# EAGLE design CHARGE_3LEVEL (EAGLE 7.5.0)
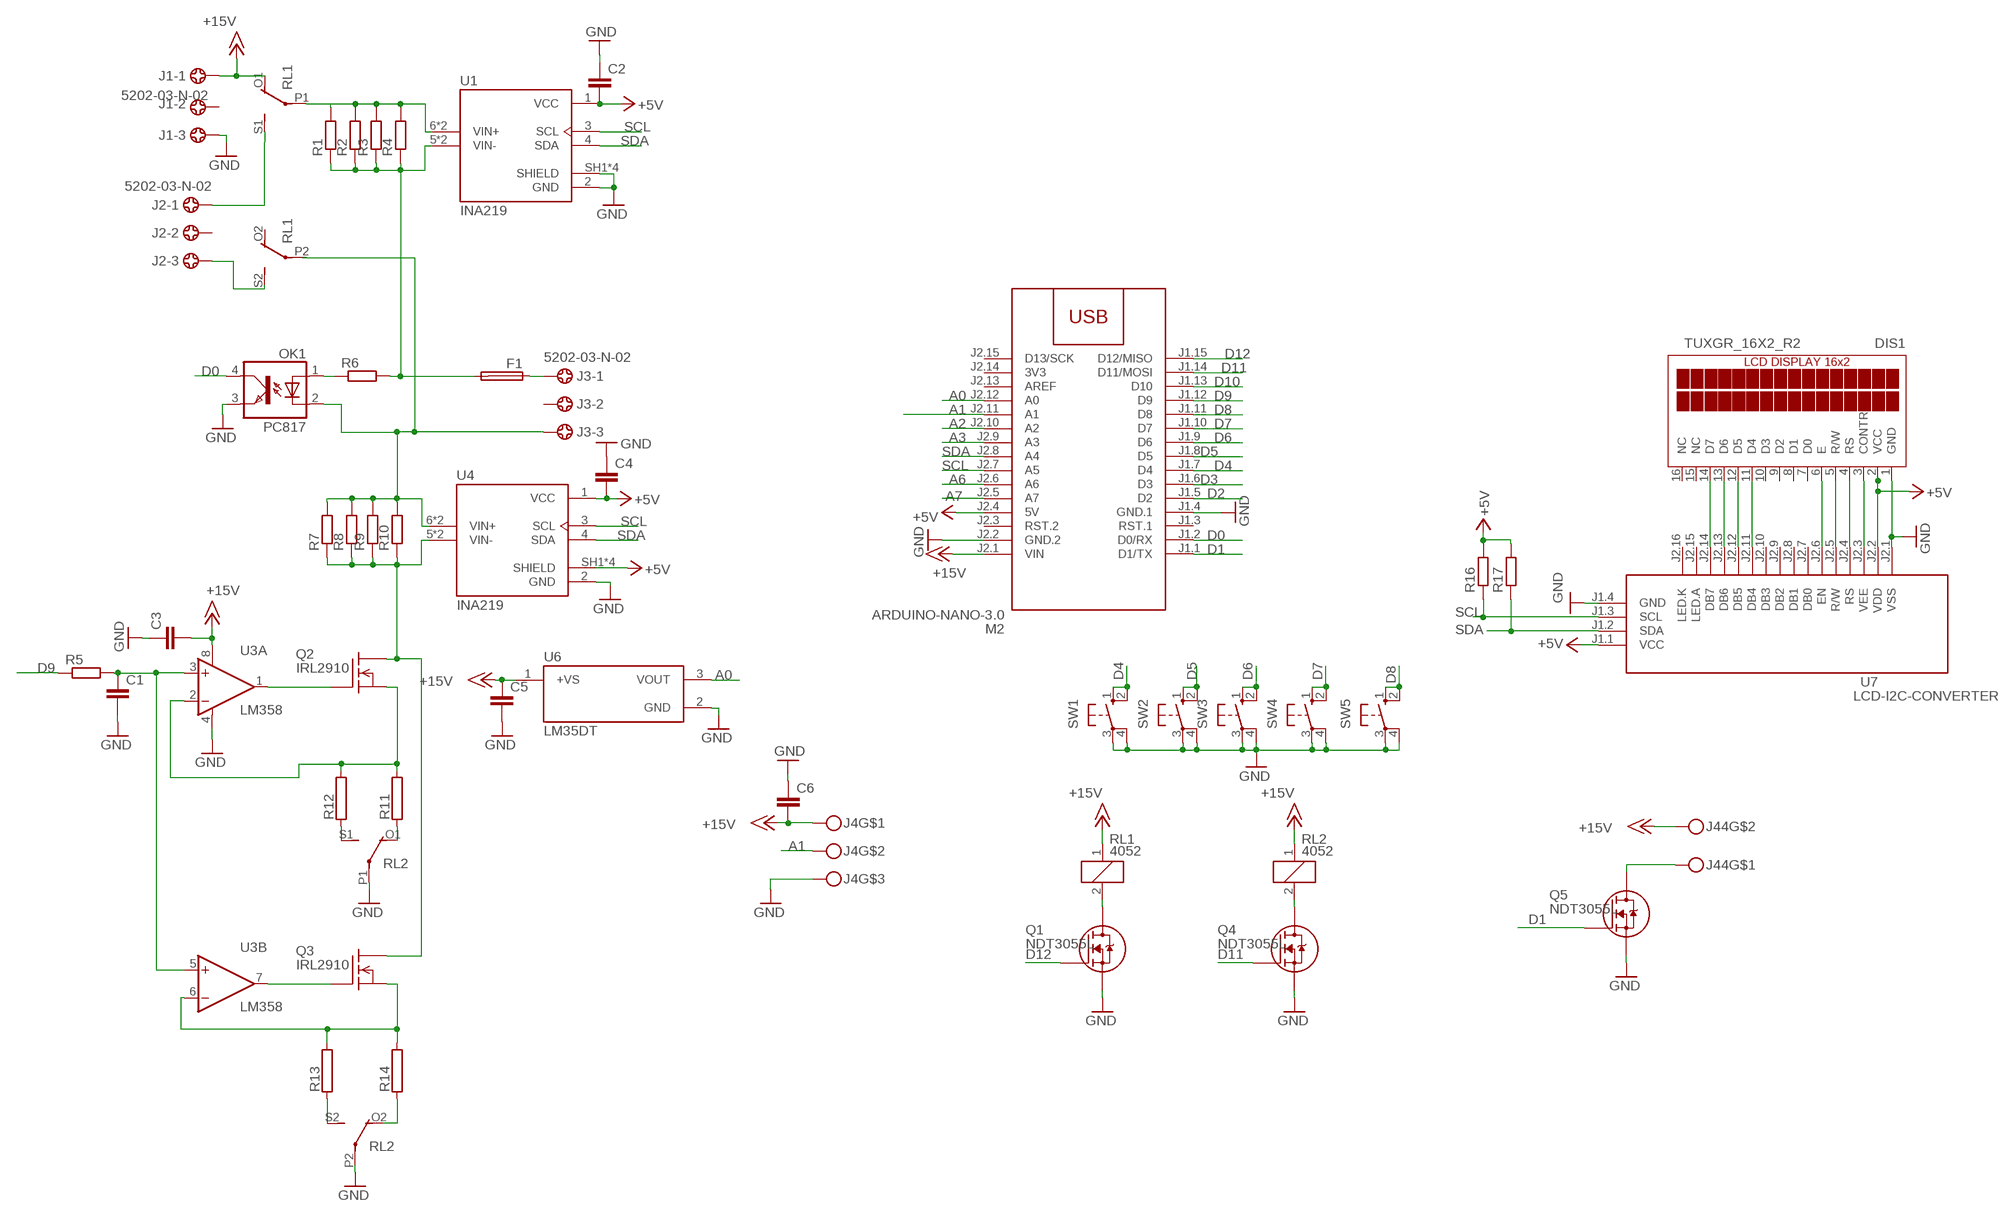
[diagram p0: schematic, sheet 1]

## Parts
C1  C-EUC1206  [C1206]
C2  C-EUC1206  [C1206]
C3  C-EUC1206  [C1206]
C4  C-EUC1206  [C1206]
C5  C-EUC1206  [C1206]
C6  C-EUC1206  [C1206]
DIS1  TUXGR_16X2_R2  [TUXGR_16X2_R2]
F1  FUSEBLANK_5X20MM  [FUSE_HOLDER_5X20MM]
J1  5202-03-N-02  [5202-03-N-02]
J2  5202-03-N-02  [5202-03-N-02]
J3  5202-03-N-02  [5202-03-N-02]
J4  MKDSN3  [MKDSN3]
J44  MKDSN1,5-2-5,08  [MKDSN1,5-2-5,08]
M2  ARDUINO-NANO-3.0  [ARDUINO-NANO-3.0]
OK1  PC817  [DIL04]
Q1  NDT3055L  [SOT223-4]
Q2  IRL2910  IRF540  [TO220]
Q3  IRL2910  IRF540  [TO220]
Q4  NDT3055L  [SOT223-4]
Q5  NDT3055L  [SOT223-4]
R1  R-EU_R2512  [R2512]
R2  R-EU_R2512  [R2512]
R3  R-EU_R2512  [R2512]
R4  R-EU_R2512  [R2512]
R5  R-EU_R1206  [R1206]
R6  R-EU_R1206  [R1206]
R7  R-EU_R2512  [R2512]
R8  R-EU_R2512  [R2512]
R9  R-EU_R2512  [R2512]
R10  R-EU_R2512  [R2512]
R11  RCA4200  [CA4200]
R12  RAC07  [AC07]
R13  RAC07  [AC07]
R14  RCA4200  [CA4200]
R16  R-EU_R1206  [R1206]
R17  R-EU_R1206  [R1206]
RL1  4052  [F4052]
RL2  4052  [F4052]
SW1  40-XX  [B3F-40XX]
SW2  40-XX  [B3F-40XX]
SW3  40-XX  [B3F-40XX]
SW4  40-XX  [B3F-40XX]
SW5  40-XX  [B3F-40XX]
U1  INA219  [MODULE_INA219]
U3  LM358  OPA2234U  [SO08]
U4  INA219  [MODULE_INA219]
U6  LM35DT  [TO254P1016X457X1955-3]
U7  LCD-I2C-CONVERTER  [LCD-I2C-CONVERTER]

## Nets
+5V: C2.2 C4.2 DIS1.2(VCC) M2.J2.4(5V) R16.2 R17.2 U1.1(VCC) U4.1(VCC) U4.SH1(SHIELD) U4.SH2(SHIELD) U4.SH3(SHIELD) U4.SH4(SHIELD) U7.J1.1(VCC) U7.J2.2(VDD)
+15V: C3.2 C5.1 C6.2 J1.1 J4.1 J44.2 M2.J2.1(VIN) RL1.1 RL1.O1(2:O) RL2.1 U3.8(A:V+) U6.1(+VS)
A0: M2.J2.12(A0) U6.3(VOUT)
A1: J4.2 M2.J2.11(A1)
A2: M2.J2.10(A2)
A3: M2.J2.9(A3)
A6: M2.J2.6(A6)
A7: M2.J2.5(A7)
D0: M2.J1.2(D0/RX) OK1.4(COL)
D1: M2.J1.1(D1/TX) Q5.1(G)
D2: M2.J1.5(D2)
D3: M2.J1.6(D3)
D4: M2.J1.7(D4) SW1.1(S) SW1.2(S1)
D5: M2.J1.8(D5) SW2.1(S) SW2.2(S1)
D6: M2.J1.9(D6) SW3.1(S) SW3.2(S1)
D7: M2.J1.10(D7) SW4.1(S) SW4.2(S1)
D8: M2.J1.11(D8) SW5.1(S) SW5.2(S1)
D9: M2.J1.12(D9) R5.1
D10: M2.J1.13(D10)
D11: M2.J1.14(D11/MOSI) Q4.1(G)
D12: M2.J1.15(D12/MISO) Q1.1(G)
GND: C1.2 C2.1 C3.1 C4.1 C5.2 C6.1 DIS1.1(GND) J1.3 J4.3 M2.J1.4(GND.1) M2.J2.2(GND.2) OK1.3(EMIT) Q1.3(S) Q4.3(S) Q5.3(S) RL2.P1(2:P) RL2.P2(3:P) SW1.3(P) SW1.4(P1) SW2.3(P) SW2.4(P1) SW3.3(P) SW3.4(P1) SW4.3(P) SW4.4(P1) SW5.3(P) SW5.4(P1) U1.2(GND) U1.SH1(SHIELD) U1.SH2(SHIELD) U1.SH3(SHIELD) U1.SH4(SHIELD) U3.4(A:V-) U4.2(GND) U6.2(GND) U7.J1.4(GND) U7.J2.1(VSS)
N$1: DIS1.14(D7) U7.J2.14(DB7)
N$2: DIS1.13(D6) U7.J2.13(DB6)
N$3: DIS1.12(D5) U7.J2.12(DB5)
N$4: DIS1.11(D4) U7.J2.11(DB4)
N$5: DIS1.6(E) U7.J2.6(EN)
N$6: DIS1.5(R/W) U7.J2.5(R/W)
N$7: DIS1.4(RS) U7.J2.4(RS)
N$8: Q2.1(G) U3.1(A:OUT)
N$9: F1.2 R1.1 R2.1 R3.1 R4.1 R6.2 U1.5(VIN-) U1.VIN-
N$10: DIS1.3(CONTR) U7.J2.3(VEE)
N$11: F1.1 J3.1
N$12: J3.3 OK1.2(C) R7.2 R8.2 R9.2 R10.2 U4.6(VIN+) U4.VIN+
N$13: OK1.1(A) R6.1
N$14: Q2.3(S) R11.2 R12.2 U3.2(A:-IN)
N$15: R13.1 RL2.S2(3:S)
N$16: Q2.2(D) Q3.2(D) R7.1 R8.1 R9.1 R10.1 U4.5(VIN-) U4.VIN-
N$17: Q3.1(G) U3.7(B:OUT)
N$18: J44.1 Q5.2(D) Q5.4(D)
N$19: C1.1 R5.2 U3.3(A:+IN) U3.5(B:+IN)
N$20: R1.2 R2.2 R3.2 R4.2 RL1.P1(2:P) U1.6(VIN+) U1.VIN+
N$21: R12.1 RL2.S1(2:S)
N$22: J2.1 RL1.S1(2:S)
N$23: J2.3 RL1.S2(3:S)
N$24: R11.1 RL2.O1(2:O)
N$25: Q3.3(S) R13.2 R14.2 U3.6(B:-IN)
N$26: R14.1 RL2.O2(3:O)
N$27: Q1.2(D) Q1.4(D) RL1.2
N$28: Q4.2(D) Q4.4(D) RL2.2
SCL: M2.J2.7(A5) R16.1 U1.3(SCL) U4.3(SCL) U7.J1.3(SCL)
SDA: M2.J2.8(A4) R17.1 U1.4(SDA) U4.4(SDA) U7.J1.2(SDA)
Unconnected: DIS1.7(D0) DIS1.8(D1) DIS1.9(D2) DIS1.10(D3) DIS1.15(NC) DIS1.16(NC) J1.2 J2.2 J3.2 M2.J1.3(RST.1) M2.J2.3(RST.2) M2.J2.13(AREF) M2.J2.15(D13/SCK) RL1.O2(3:O) RL1.P2(3:P) U7.J2.7(DB0) U7.J2.8(DB1) U7.J2.9(DB2) U7.J2.10(DB3) U7.J2.15(LED.A) U7.J2.16(LED.K)

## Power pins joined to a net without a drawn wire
3V3: M2.J2.14(3V3)

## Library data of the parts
C1-C6 = rcl:C-EU: CAPACITOR, European symbol
DIS1 = display-lcd:TUXGR_16X2_R2: Tuxgraphics LCD display 16x2 characters reflective, without background light Source: tuxgr_12x2_r2.pdf; OC_FARNELL: unknown; OC_NEWARK: unknown
F1 = fuse:FUSE: Fuse; OC_FARNELL: unknown; OC_NEWARK: unknown
J1-J3 = con-ebyelectro:5202-03-N-02: Barrier Blocks Sreies 5202 Source: http://www.ebyelectro.com/PDF/5202-XX-N-02.pdf; OC_FARNELL: unknown; OC_NEWARK: unknown
J4 = con-phoenix-508:MKDSN3
J44 = con-phoenix-508:MKDSN1,5-2-5,08
M2 = diy-modules:ARDUINO-NANO-3.0: Arduino Nano 3.0 and compatible devices More details available here: https://www.arduino.cc/en/Main/ArduinoBoardNano Click here to find device on ebay.com
OK1 = optocoupler:PC817: SHARP OPTO COUPLER; MPN: PC817X4J000F; OC_FARNELL: 9707727; OC_NEWARK: 97K7059
Q1 Q4 Q5 = NDT3055L:NDT3055L: Trans MOSFET N-CH 60V 4A 4-Pin(3+Tab) SOT-223 Trans MOSFET N-CH 60V 4A 4-Pin(3+Tab) SOT-223 Check availability; AVAILABILITY: In Stock; CHECK_PRICES: https://www.snapeda.com/parts/NDT3055L/Onsemi/view-part/?ref=eda; DESCRIPTION: Trans MOSFET N-CH 60V 4A 4-Pin(3+Tab) SOT-223 Trans MOSFET N-CH 60V 4A 4-Pin(3+Tab) SOT-223; MF: ON; MP: NDT3055L; PACKAGE: SOT-223-4 Fairchild Semiconductor; PRICE: None; SNAPEDA_LINK: https://www.snapeda.com/parts/NDT3055L/Onsemi/view-part/?ref=snap
Q2 Q3 = transistor-fet:IRF540: N-Channel Enhancement MOSFET (HEXFET); 100V; 28A; 0,077Ohm
R1-R10 R16 R17 = rcl:R-EU_: RESISTOR, European symbol
R11-R14 = resistor-power:R: Power Resitor; OC_FARNELL: unknown; OC_NEWARK: unknown
RL1 RL2 = relay:4052: RELAY 2 x switch, Finder; OC_FARNELL: unknown; OC_NEWARK: unknown
SW1-SW5 = switch-omron:40-XX: OMRON SWITCH; MF: OMRON COMPONENTS USA; MPN: B3F-4000; OC_FARNELL: 176434; OC_NEWARK: 36K3105
U1 U4 = INA219:INA219: Check availability; AVAILABILITY: Not in stock; CHECK_PRICES: https://www.snapeda.com/parts/INA219%20High%20Side%20DC%20Current%20Sensor%20Breakout%20-%2026V%20%C2%B13.2A%20Max%20-%20STEMMA%20QT/Adafruit+Industries/view-part/?ref=eda; DESCRIPTION: INA219 High Side DC Current Sensor Breakout - 26V ±3.2A Max | Adafruit Industries 904; MF: Adafruit Industries; MP: INA219 High Side DC Current Sensor Breakout - 26V ±3.2A Max - STEMMA QT; PACKAGE: NON-STANDARD-8 ADAFRUIT; PRICE: None; SNAPEDA_LINK: https://www.snapeda.com/parts/INA219%20High%20Side%20DC%20Current%20Sensor%20Breakout%20-%2026V%20%C2%B13.2A%20Max%20-%20STEMMA%20QT/Adafruit+Industries/view-part/?ref=snap
U3 = burr-brown:OPA2234: Operational Amplifier; MF: TEXAS INSTRUMENTS; MPN: OPA2234U; OC_FARNELL: 1212441; OC_NEWARK: 96K4523
U6 = LM35DT-H:LM35DT: Check availability; AVAILABILITY: In Stock; CHECK_PRICES: https://www.snapeda.com/parts/LM35DT/Texas+Instruments/view-part/?ref=eda; DESCRIPTION: ±0.5°C 4V-30V, Temperature sensor with analog output 3-TO-220 0 to 100; MF: Texas Instruments; MP: LM35DT; PACKAGE: TO-220-3 Texas Instruments; PRICE: None; SNAPEDA_LINK: https://www.snapeda.com/parts/LM35DT/Texas+Instruments/view-part/?ref=snap
U7 = diy-modules:LCD-I2C-CONVERTER: I2C Bus to 4-Bit Parallel LCD Interface with LED backlight driver

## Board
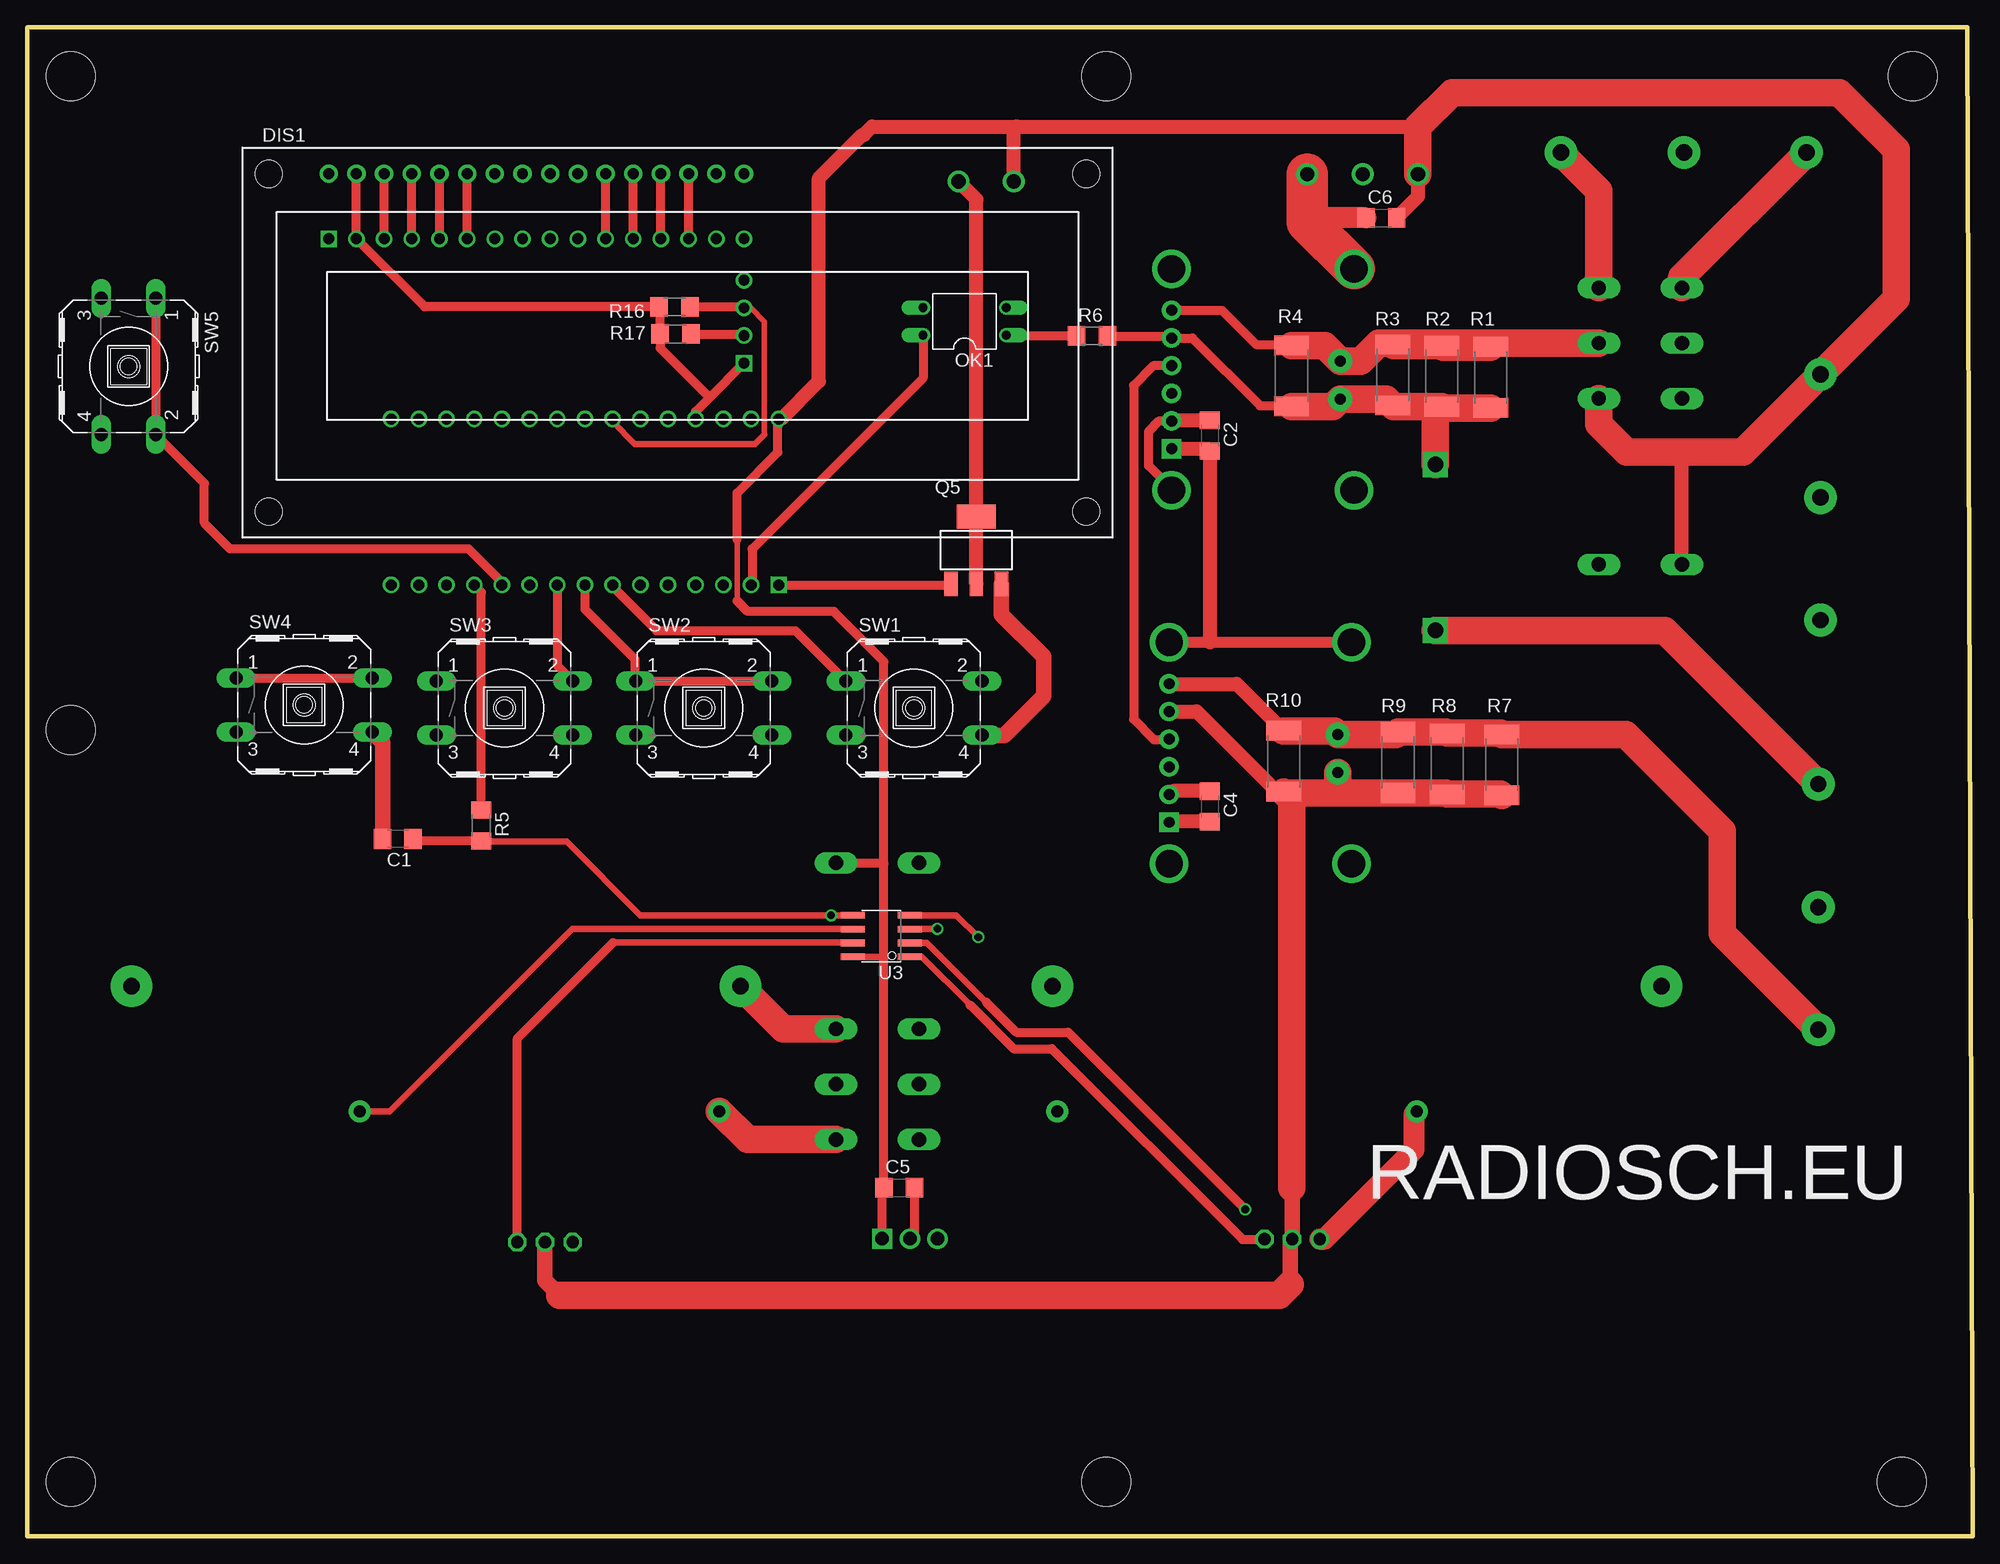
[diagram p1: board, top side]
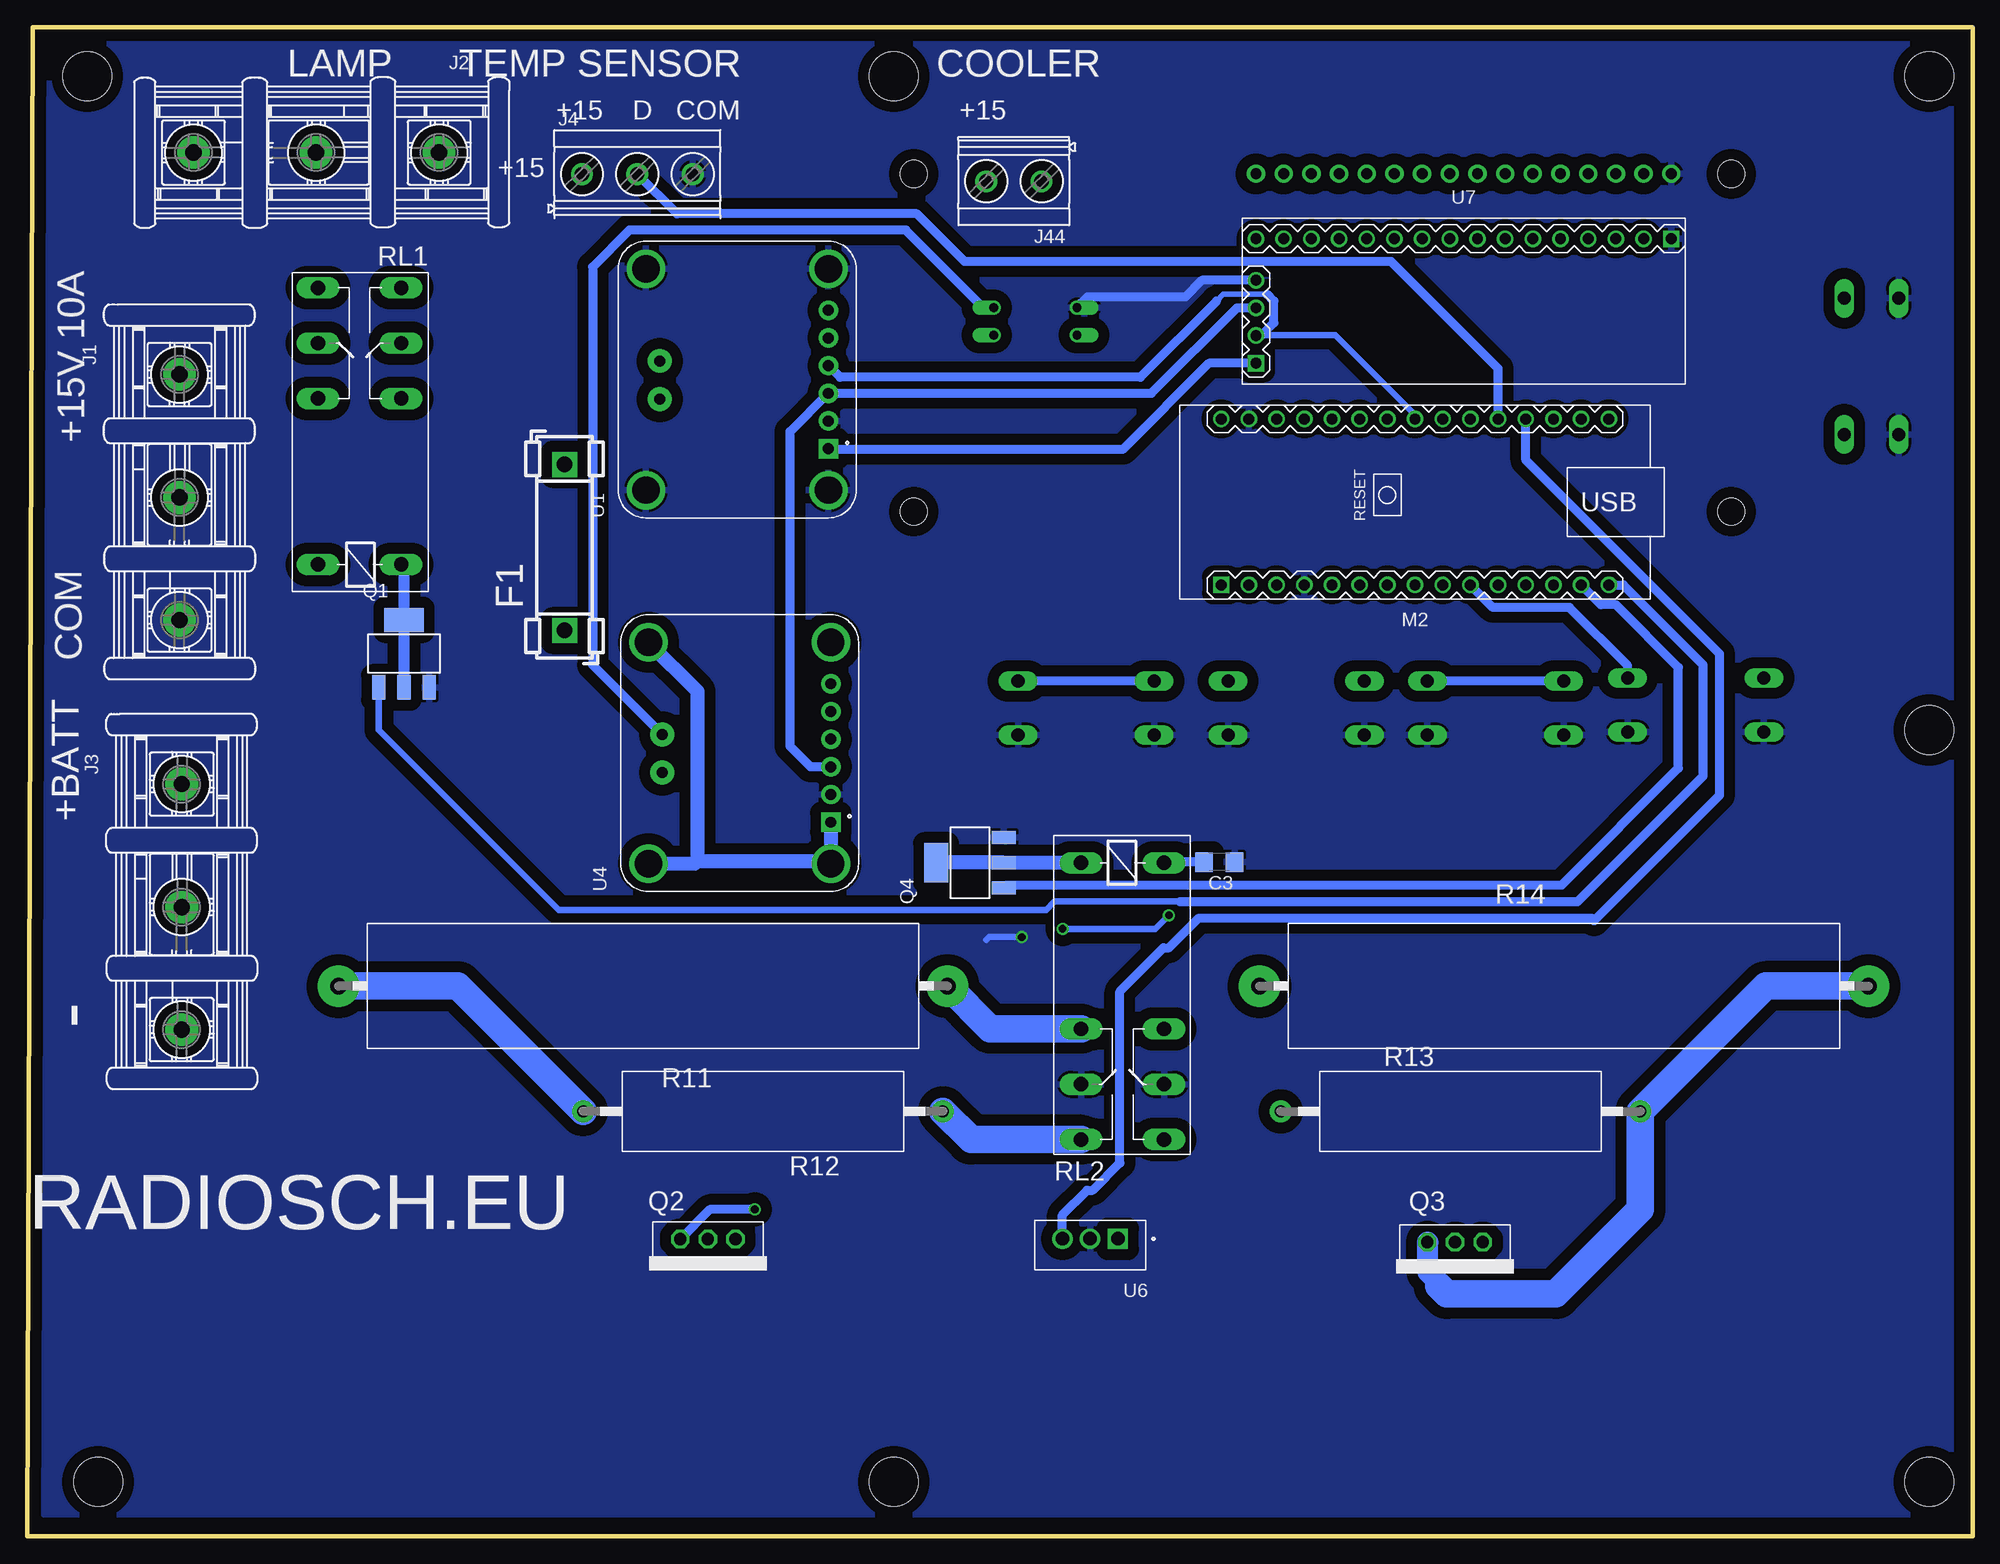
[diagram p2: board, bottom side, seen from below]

Size 178.5 x 138.5 mm. Coordinates in mm from the lower left corner, seen from the top.
Outline: 0,0 178.5,0 178,138.5 0,138.5 0,0
Copper layers (1*16): Top 0.035mm / dielectric 1.5mm / Bottom 0.035mm
Design rules "default": minimum track width 10mil, minimum drill 24mil, track to track 8mil, track to pad 8mil, pad to pad 8mil, via to via 8mil, smd to smd 8mil, copper to edge 40mil, drill to drill 8mil, minimum pad ring 10mil, minimum via ring 8mil, stop-mask expansion 4mil, vias tented up to drill 0mil, thermal gap 10mil
Holes 4.5 mm at 4,134 4,74 4,5 99,5 172,5 173,134 99,134

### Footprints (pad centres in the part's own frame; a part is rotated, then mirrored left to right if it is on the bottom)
C1206 = smd 1.6 x 1.8: 1 -1.4,0; 2 1.4,0
TUXGR_16X2_R2 = drill 1 pad 1.676: 1 -32,15.5; 2 -29.46,15.5; 3 -26.92,15.5; 4 -24.38,15.5; 5 -21.84,15.5; 6 -19.3,15.5; 7 -16.76,15.5; 8 -14.22,15.5; 9 -11.68,15.5; 10 -9.14,15.5; 11 -6.6,15.5; 12 -4.06,15.5; 13 -1.52,15.5; 14 1.02,15.5; 15 3.56,15.5; 16 6.1,15.5 | hole 2.5: -37.5,-15.5; 37.5,-15.5; -37.5,15.5; 37.5,15.5
FUSE_HOLDER_5X20MM = drill 1.422 pad 2.286 square: 1 0,0; 2 15.24,0
5202-03-N-02 = drill 1.5 pad 3: 1 -9.29,0; 2 2,0; 3 13.25,0
MKDSN3 = drill 1.3 pad 2: 1 -5.101,0.025; 2 -0.021,0.025; 3 5.059,0.025
MKDSN1,5-2-5,08 = drill 1.3 pad 2: 1 -2.561,0.025; 2 2.519,0.025
ARDUINO-NANO-3.0 = drill 1 square: J1.1 17.78,7.62 | drill 1: J1.2 15.24,7.62; J1.3 12.7,7.62; J1.4 10.16,7.62; J1.5 7.62,7.62; J1.6 5.08,7.62; J1.7 2.54,7.62; J1.8 0,7.62; J1.9 -2.54,7.62; J1.10 -5.08,7.62; J1.11 -7.62,7.62; J1.12 -10.16,7.62; J1.13 -12.7,7.62; J1.14 -15.24,7.62; J1.15 -17.78,7.62; J2.1 17.78,-7.62; J2.2 15.24,-7.62; J2.3 12.7,-7.62; J2.4 10.16,-7.62; J2.5 7.62,-7.62; J2.6 5.08,-7.62; J2.7 2.54,-7.62; J2.8 0,-7.62; J2.9 -2.54,-7.62; J2.10 -5.08,-7.62; J2.11 -7.62,-7.62; J2.12 -10.16,-7.62; J2.13 -12.7,-7.62; J2.14 -15.24,-7.62; J2.15 -17.78,-7.62
DIL04 = drill 0.813 offset: 1 -1.27,-3.81; 2 1.27,-3.81; 3 1.27,3.81; 4 -1.27,3.81
SOT223-4 = smd 1.219 x 2.235: 1 -2.24,-3.091; 2 0.071,-3.091; 3 2.383,-3.091 | smd 3.6 x 2.2: 4 0.071,3.107
TO220 = drill 1.118 octagon: 1 -2.54,0; 2 0,0; 3 2.54,0
R2512 = smd 1.8 x 3.2: 1 -2.8,0; 2 2.8,0
R1206 = smd 1.6 x 1.803: 1 -1.422,0; 2 1.422,0
CA4200 = drill 1.5 pad 3.81: 1 -27.94,0; 2 27.94,0
AC07 = drill 1.1 pad 2: 1 -16.5,0; 2 16.5,0
F4052 = drill 1.321 long: 1 -3.81,3.81; 2 -3.81,-3.81; O1 11.43,-3.81; O2 11.43,3.81; P1 16.51,-3.81; P2 16.51,3.81; S1 21.59,-3.81; S2 21.59,3.81
B3F-40XX = drill 1.194 long: 1 -6.248,2.489; 2 6.248,2.489; 3 -6.248,-2.489; 4 6.248,-2.489
MODULE_INA219 = drill 1 pad 1.778 square: 1 -6.35,-9.12 | drill 1 pad 1.778: 2 -3.81,-9.12; 3 -1.27,-9.12; 4 1.27,-9.12; 5 3.81,-9.12; 6 6.35,-9.12 | drill 2.5 pad 3.2: SH1 -10.16,7.62; SH2 10.16,7.62; SH3 -10.16,-9.12; SH4 10.16,-9.12 | drill 1 pad 2.184: VIN+ 1.7,6.35; VIN- -1.8,6.35
SO08 = smd 0.61 x 2.21: 1 -1.905,-2.616; 2 -0.635,-2.616; 3 0.635,-2.616; 4 1.905,-2.616; 5 1.905,2.616; 6 0.635,2.616; 7 -0.635,2.616; 8 -1.905,2.616
TO254P1016X457X1955-3 = drill 1.24 square: 1 -2.54,-0.573 | drill 1.24: 2 0,-0.573; 3 2.54,-0.573
LCD-I2C-CONVERTER = drill 1 square: J1.1 -19.05,-5.08; J2.1 19.05,6.35 | drill 1: J1.2 -19.05,-2.54; J1.3 -19.05,0; J1.4 -19.05,2.54; J2.2 16.51,6.35; J2.3 13.97,6.35; J2.4 11.43,6.35; J2.5 8.89,6.35; J2.6 6.35,6.35; J2.7 3.81,6.35; J2.8 1.27,6.35; J2.9 -1.27,6.35; J2.10 -3.81,6.35; J2.11 -6.35,6.35; J2.12 -8.89,6.35; J2.13 -11.43,6.35; J2.14 -13.97,6.35; J2.15 -16.51,6.35; J2.16 -19.05,6.35

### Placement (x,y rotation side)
C1  34,64 180 top
C2  108.5,101 270 top
C3  69.12,61.88 180 bottom
C4  108.5,67 270 top
C5  80,32 0 top
C6  124.25,121 0 top
DIS1  59.66,109.55 0 top
F1  129.2,83.13 90 bottom
J1  164.53,97.34 270 bottom
J2  150,127 180 bottom
J3  164.33,59.75 270 bottom
J4  122.5,125 0 bottom
J44  88,124.38 180 bottom
M2  51.17,94.93 180 bottom
OK1  86,111.5 90 top
Q1  144,81 0 bottom
Q2  116.05,27.27 180 bottom
Q3  47.5,27 180 bottom
Q4  92,61.75 90 bottom
Q5  87,90.5 0 top
R1  134.27,106.36 90 top
R2  129.77,106.47 90 top
R3  125.27,106.58 90 top
R4  116,106.5 90 top
R5  41.66,65.24 270 top
R6  97.68,110.16 0 top
R7  135.27,70.8 90 top
R8  130.27,70.91 90 top
R9  125.77,71.02 90 top
R10  115.27,71.13 90 top
R11  122,50.5 180 bottom
R12  111,39 180 bottom
R13  47,39 0 bottom
R14  37.5,50.5 0 bottom
R16  59.4,112.84 180 top
R17  59.48,110.34 180 top
RL1  148,93 90 bottom
RL2  78,58 270 bottom
SW1  81.35,76.02 0 top
SW2  62.07,76.02 0 top
SW3  43.79,76.02 0 top
SW4  25.41,76.3 0 top
SW5  9.3,107.37 270 top
U1  114.11,106.17 90 bottom
U3  78.35,55.09 90 top
U4  113.89,71.89 90 bottom
U6  80.98,26.73 180 bottom
U7  46.71,112.74 0 bottom

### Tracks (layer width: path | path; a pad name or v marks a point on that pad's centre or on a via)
+5V
  Top 0.813: M2.J2.4 61.33,103.23 62.61,104.51 | 62.61,104.51 U7.J1.1 | 62.61,104.51 58.06,109.07 R17.2 58.06,112.76 R16.2 36.45,112.84 U7.J2.2 DIS1.2
  Top 1.016: U4.SH2 108.5,82.05 U4.SH4
  Top 1.27: C4.2 104.83,65.6 U4.1 | 108.5,82.05 C2.2 108.28,99.82 U1.1
  Bottom 0.813: U7.J1.1 70.09,107.66 78,99.75 104.92,99.75 U1.1
  Bottom 1.27: U4.1 U4.SH3 105.04,62 117,62 | U4.SH1 117.27,61.73 117,62 | 117,62 117,77.54 U4.SH2
+15V
  Top 0.5: 65.12,85.88 65.12,91.5
  Top 0.61: U3.8 78.42,53.19 78.6,53
  Top 0.813: 65.12,85.88 66.12,84.88 74,84.88 78.6,80.28 78.6,61.75 | 65.12,91.5 65.12,95.75 68.88,99.5 68.88,102.47 M2.J2.1 | U6.1 78.44,31.84 C5.1 78.6,53 78.6,61.75 | RL2.1 78.54,61.81 78.6,61.75
  Top 1.27: M2.J2.1 69.17,102.55 72.62,106 72.62,124.62 76.62,128.62 76.75,128.62 77.5,129.38 90.75,129.38 | 90.75,129.38 127.58,129.38 127.6,129.35 | J44.2 90.52,129.14 90.75,129.38 | RL1.1 151.81,99.31 152,99.5 | J4.1 127.6,122.95 C6.2
  Top 2.54: RL1.O1 144.19,102.06 146.75,99.5 152,99.5 157.4,99.5 J1.1 171.5,113.6 171.5,127.25 166.25,132.5 130.75,132.5 127.6,129.35 J4.1
  Bottom 0.813: C3.2 74.12,61.88 RL2.1
A0
  Bottom 0.813: U6.3 83.52,29.48 81.25,31.75 80.75,31.75 78.25,34.25 78.25,50 74.25,54 73.75,54 71,56.75 35,56.75 34.75,56.5 23.25,68 23.25,81 41,98.75 M2.J2.12
A1
  Bottom 0.813: M2.J2.11 43.55,107.17 53.38,117 92.5,117 96.88,121.38 118.87,121.38 J4.2
D0
  Top 0.813: OK1.4 82.19,106.31 66.5,90.62 66.5,87.4 M2.J1.2
D1
  Top 0.813: M2.J1.1 84.66,87.31 Q5.1
D4
  Top 0.813: M2.J1.7 53.71,87.17 57.75,83.12 70.49,83.12 SW1.1
  Bottom 0.813: SW1.1 SW1.2
D5
  Top 0.813: M2.J1.8 51.17,85.08 55.75,80.5 55.75,78.58 SW2.1 SW2.2
D6
  Top 0.813: M2.J1.9 48.63,79.92 SW3.2
  Bottom 0.813: SW3.1 SW3.2
D7
  Top 0.813: SW4.1 SW4.2
  Bottom 0.813: SW4.2 31.66,79.91 37,85.25 44.03,85.25 M2.J1.10
D8
  Top 0.813: SW5.1 SW5.2 16.25,96.66 16.25,93 18.62,90.62 40.5,90.62 43.55,87.58 M2.J1.11
D9
  Top 0.813: R5.1 41.66,86.66 M2.J1.12
D11
  Bottom 0.61: 88.67,59.75 Q4.1
  Bottom 0.813: 88.67,59.75 37.75,59.75 27,70.5 27,79.75 32.75,85.5 34.12,85.5 M2.J1.14
D12
  Bottom 0.61: 72.75,58.25 84.25,58.25 85,57.5 129.75,57.5 146.24,73.99 Q1.1
  Bottom 0.813: M2.J1.15 32.06,87.31 24.75,80 24.75,69.75 36.25,58.25 72.75,58.25
GND  (via drill 0.7)
  Top 0.61: U3.4 85.25,56.99 v87.25,55
  Top 0.813: U1.SH3 104.99,96.14 102.88,98.25 102.88,101.38 103.88,102.38 104.97,102.38 U1.2 | C5.2 81.4,27.72 U6.2
  Top 1.27: C4.1 105.09,68.4 U4.2 | C2.1 105.03,102.4 U1.2
  Top 1.422: Q5.3 89.38,84.62 93.25,80.75 93.25,77.12 89.62,73.5 87.63,73.5 SW1.4 | C1.2 32.6,72.87 SW4.4
  Top 1.93: C6.1 118.94,121 117.44,122.5
  Top 3.81: J4.3 117.44,122.5 117.44,120.62 U1.SH2
  Bottom 0.61: v87.25,55 90.25,55 90.5,54.75
  Bottom 0.813: U7.J1.4 70.72,115.28 72.25,113.75 81.21,113.75 OK1.3
  pour Bottom (isolate 1.016): 2,137 177,137 177,2 2,2
N$1
  Top 0.813: U7.J2.14 DIS1.14
N$2
  Top 0.813: U7.J2.13 DIS1.13
N$3
  Top 0.813: U7.J2.12 DIS1.12
N$4
  Top 0.813: U7.J2.11 DIS1.11
N$5
  Top 0.813: U7.J2.6 DIS1.6
N$6
  Top 0.813: DIS1.5 U7.J2.5
N$7
  Top 0.813: U7.J2.4 DIS1.4
N$8
  Top 0.61: U3.1 82.06,53.19 86.5,48.75
  Top 0.813: Q2.1 113.49,27.25 111.5,27.25 94,44.75 90.5,44.75 86.5,48.75
N$9
  Top 0.813: R6.2 104.81,110.16 U1.5 106.89,109.98 113.12,103.75 115.95,103.75 R4.1
  Top 2.54: R1.1 129.88,103.56 R2.1 | R2.1 125.38,103.67 R3.1 124.68,104.37 U1.VIN- 119.79,103.7 R4.1 | F1.2 129.2,103.1 R2.1
N$10
  Top 0.813: U7.J2.3 DIS1.3
N$11
  Top 2.54: F1.1 150.24,83.13 J3.1
N$12
  Top 1.27: U4.6 110.96,78.24 R10.2
  Top 2.54: R10.2 119.9,73.93 U4.VIN+ 125.54,73.59 R9.2 130.16,73.82 R8.2 135.16,73.71 R7.2 146.65,73.6 155.5,64.75 155.5,55.33 J3.3
  Bottom 0.5: 125.62,78.97 U4.VIN+
  Bottom 0.813: OK1.2 90.77,112.77 97.88,119.88 123.25,119.88 126.62,116.5 126.62,79.97 U4.VIN+
N$13
  Top 0.813: R6.1 89.88,110.16 OK1.1
N$14  (via drill 0.7)
  Top 0.61: U3.2 82.55,54.45 88,49
  Top 0.813: 88,49 90.75,46.25 95.5,46.25 v111.75,30
  Top 1.93: Q2.3 119.02,27.27 127.25,35.5 127.25,38.75 R12.2
  Bottom 0.813: v111.75,30 115.86,30 Q2.3
  Bottom 2.54: R11.2 139,50.5 R12.2
N$15
  Top 2.54: RL2.S2 66.09,36.41 R13.1
N$16
  Top 1.27: U4.5 107.3,75.7 114.5,68.5 115.1,68.5 R10.1
  Top 1.422: 116,32 116.05,31.95 Q2.2 115.88,27.09 115.88,23.12 | Q3.2 47.5,23.5 48.88,22.12
  Top 2.54: 120.5,68.22 R9.1 130.16,68.22 R8.1 135.16,68.11 R7.1 | 120.5,68.22 115.38,68.22 R10.1 116,67.6 116,32 | U4.VIN- 120.24,68.48 120.5,68.22 | 48.88,22.12 114.88,22.12 115.88,23.12
N$17
  Top 0.61: 53.75,54.5 75.69,54.5 U3.7
  Top 0.813: Q3.1 44.96,45.71 53.75,54.5
N$18
  Top 1.27: J44.1 87.07,122.72 Q5.4 Q5.2
N$19  (via drill 0.7)
  Top 0.61: U3.3 83.47,55.73 v83.5,55.75 | U3.5 v73.75,56.99 56.26,56.99 49.5,63.75 41.73,63.75 R5.2
  Top 0.813: R5.2 35.58,63.82 C1.1
  Bottom 0.61: v83.5,55.75 75,55.75 v73.75,56.99
N$20
  Top 0.813: U1.6 109.61,112.52 112.75,109.38 115.92,109.38 R4.2
  Top 2.54: R1.2 129.88,109.16 R2.2 125.38,109.27 R3.2 125.15,109.5 124.75,109.5 | R4.2 119.03,109.3 U1.VIN+ 122.37,107.87 124,109.5 124.75,109.5 | RL1.P1 124.76,109.51 124.75,109.5
N$21
  Bottom 2.54: RL2.S1 91.91,36.41 R12.1
N$22
  Top 2.54: RL1.S1 144.19,123.52 J2.1
N$23
  Top 2.54: RL1.S2 151.81,115.56 J2.3
N$24
  Bottom 2.54: RL2.O1 90.13,46.57 R11.1
N$25
  Top 0.61: U3.6 75.71,55.75 50,55.75 33.25,39 R13.2
  Bottom 1.93: 49,23 49,23.25 50,24.25 50,26.96 Q3.3
  Bottom 2.54: 49,23 48.25,22.25 38.25,22.25 30.5,30 R13.2 19,50.5 R14.2
N$26
  Top 2.54: RL2.O2 69.37,46.57 R14.1
N$27
  Bottom 1.016: Q1.2 Q1.4 143.93,88.93 RL1.2
N$28
  Bottom 1.27: RL2.2 88.9,61.81 Q4.2 Q4.4
SCL
  Top 0.5: 67.62,101.12 67.62,111.5 66.38,112.75 U7.J1.3
  Top 0.61: M2.J2.7 53.71,102.29 55.75,100.25 66.75,100.25 67.62,101.12
  Top 0.813: R16.1 65.66,112.84 U7.J1.3
  Bottom 0.813: U4.3 106.62,70.62 108.5,72.5 108.5,101.39 U1.3 75.35,104.9 67.5,112.75 U7.J1.3
SDA
  Top 0.813: U1.4 103.31,107.44 101.5,105.62 101.5,75 103.38,73.12 104.73,73.12 U4.4 | R17.1 65.62,110.34 U7.J1.2
  Bottom 0.5: 64.75,114 68.75,114 69.38,113.38
  Bottom 0.61: M2.J2.8 51.17,102.92 58.5,110.25 65.71,110.25 U7.J1.2
  Bottom 0.813: U7.J1.2 65.3,110.2 64.12,111.38 64.12,113.38 64.75,114 | 69.38,113.38 76.38,106.38 103.92,106.38 U1.4

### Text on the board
tNames: RADIOSCH.EU
bNames: COOLER | TEMP SENSOR | LAMP | +15 | COM | D | +15 | +15 | +15V 10A | COM | +BATT | - | RADIOSCH.EU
